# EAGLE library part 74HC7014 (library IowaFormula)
Hex BUFFER, non-inverting Google Drive Datasheet
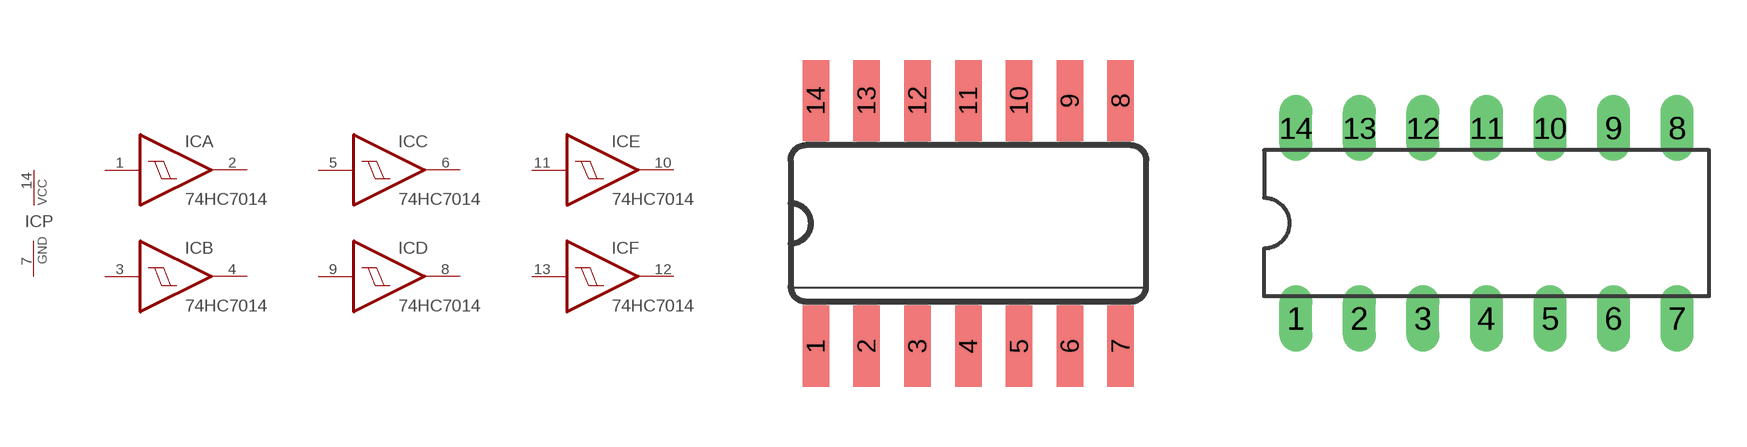
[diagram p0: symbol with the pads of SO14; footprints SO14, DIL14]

Designator prefix IC; gates P=PWR A=7417 B=7417 C=7417 D=7417 E=7417 F=7417

## 74HC7014  [SO14]
1  A:I  in
2  A:O  out
3  B:I  in
4  B:O  out
5  C:I  in
6  C:O  out
7  P:GND  pwr
8  D:O  out
9  D:I  in
10  E:O  out
11  E:I  in
12  F:O  out
13  F:I  in
14  P:VCC  pwr

## 74HC7014DIL14  [DIL14]
Pads as for SO14

## Footprint SO14 (pad centres in mm)
Small Outline package 150 mil
smd 0.66 x 2.032: 1 -3.81,-3.073; 2 -2.54,-3.073; 3 -1.27,-3.073; 4 0,-3.073; 5 1.27,-3.073; 6 2.54,-3.073; 7 3.81,-3.073; 8 3.81,3.073; 9 2.54,3.073; 10 1.27,3.073; 11 0,3.073; 12 -1.27,3.073; 13 -2.54,3.073; 14 -3.81,3.073

## Footprint DIL14 (pad centres in mm)
Dual In Line Package
drill 0.813 long: 1 -7.62,-3.81; 2 -5.08,-3.81; 3 -2.54,-3.81; 4 0,-3.81; 5 2.54,-3.81; 6 5.08,-3.81; 7 7.62,-3.81; 8 7.62,3.81; 9 5.08,3.81; 10 2.54,3.81; 11 0,3.81; 12 -2.54,3.81; 13 -5.08,3.81; 14 -7.62,3.81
